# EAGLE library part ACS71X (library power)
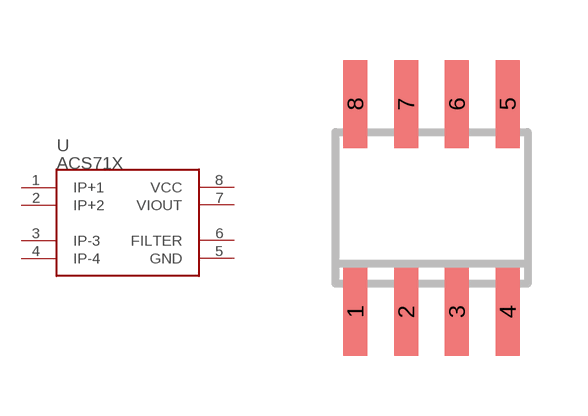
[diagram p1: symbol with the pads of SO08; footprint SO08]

Designator prefix U

## ACS71X  [SO08]
1  IP+1
2  IP+2
3  IP-3
4  IP-4
5  GND
6  FILTER
7  VIOUT
8  VCC

## Footprint SO08 (pad centres in mm)
SMALL OUTLINE INTEGRATED CIRCUIT body 3.9 mm/JEDEC MS-012AA
smd 0.6 x 2.2: 1 -1.905,-2.6; 2 -0.635,-2.6; 3 0.635,-2.6; 4 1.905,-2.6; 5 1.905,2.6; 6 0.635,2.6; 7 -0.635,2.6; 8 -1.905,2.6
